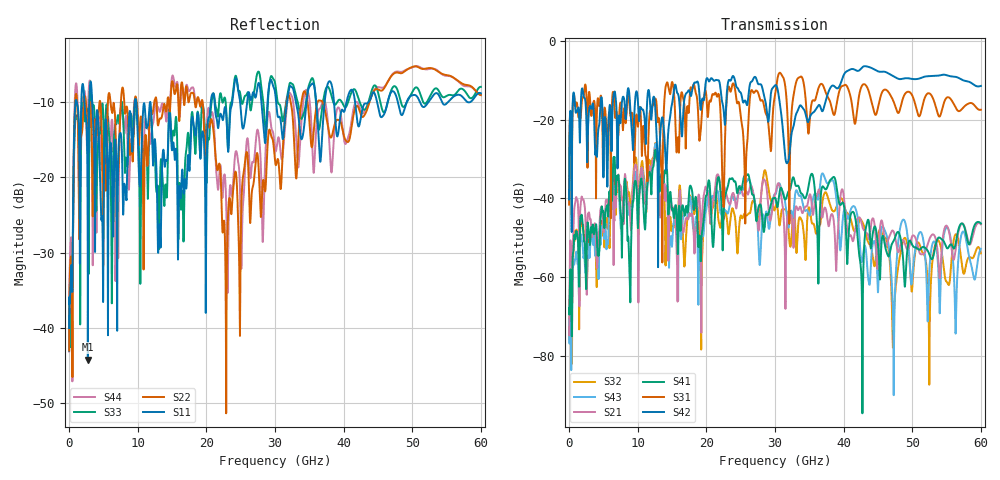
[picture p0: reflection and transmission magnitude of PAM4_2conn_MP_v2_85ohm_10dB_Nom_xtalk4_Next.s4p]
! Info: Touchstone file created by Circ.  Input file=FAB50GbE_2conn_Midplane_Examax_Topo2_v2_85ohm_10dB_Nom.circ
# Hz S RI R 50
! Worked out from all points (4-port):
!   6000 points, 10 MHz to 60 GHz, reference 50 ohm
!   strongest paths, dB at 10 MHz, 15.01 GHz, 30.01 GHz, 45.01 GHz, 60 GHz:
!     S42: -40.2, -15.9, -11.3, -7.7, -11.4
!     S31: -41.6, -10.4, -13.7, -16.9, -17.5
!     S41: -67.8, -42.8, -39.8, -51.8, -46.3
!     S21: -74.8, -43.2, -38.9, -55.9, -46.6
!     S43: -70.7, -52.0, -39.0, -63.9, -52.8
!     S32: -74.2, -47.3, -42.6, -49.7, -53.9
!   lowest |S11| = -44.2 dB at 2.74 GHz (marker M1), VSWR 1.01, Z = 49.7 + j0.52 ohm
!   |S11| at or under -10 dB: 3.366 GHz to 9.579 GHz (6.213 GHz wide, 96 % of centre); 11.83 GHz to 20.65 GHz (8.822 GHz wide, 54.3 % of centre); 21.2 GHz to 23.79 GHz (2.59 GHz wide, 11.5 % of centre)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
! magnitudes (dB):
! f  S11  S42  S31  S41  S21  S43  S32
! 10 MHz  -40.0  -40.2  -41.6  -67.8  -74.8  -70.7  -74.2
! 2.74 GHz  -44.2  -23.5  -21.8  -46.3  -44.1  -53.7  -52.0
! 12.63 GHz  -16.6  -19.3  -14.7  -27.9  -28.4  -26.2  -26.1
! 19.24 GHz  -16.1  -16.8  -21.6  -52.9  -58.1  -49.2  -76.1
! 28.55 GHz  -15.4  -14.8  -17.8  -45.9  -35.5  -46.2  -32.8
! 47.25 GHz  -8.6  -8.9  -15.3  -50.9  -48.3  -75.6  -73.9
! 60 GHz  -8.9  -11.4  -17.5  -46.3  -46.6  -52.8  -53.9
